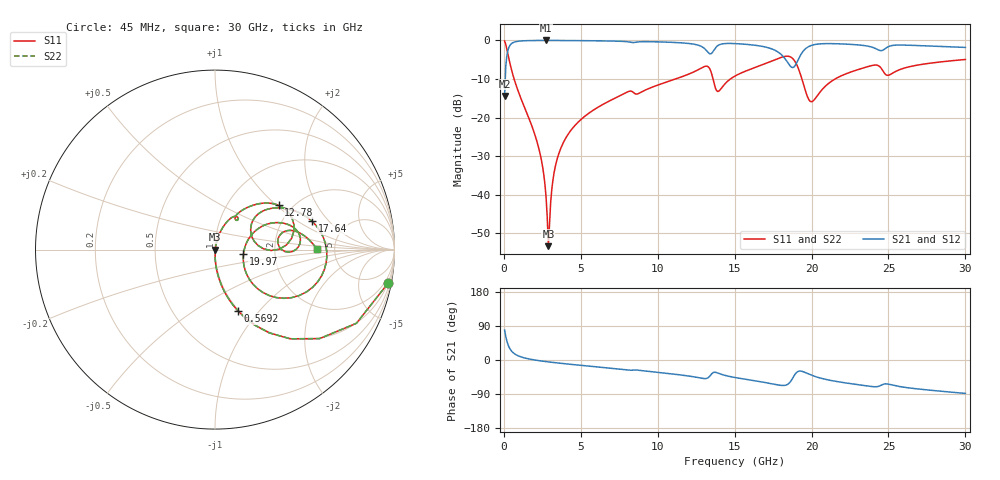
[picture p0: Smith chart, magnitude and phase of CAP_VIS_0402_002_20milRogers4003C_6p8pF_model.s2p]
! S-parameter model data by Modelithics Inc.  support@modelithics.com  813-866-6335  Tampa FL USA
! S-Parameter data specifications:
! Substrate: 20-mil Rogers 4003C, substrate thickness, H=0.508mm, Dielectric constant, Er=3.75
! PCB Mounting Pad Footprint: Pad width, PadW=0.50mm , Pad length, PadL=0.50mm , Pad gap, PadG (edge-to-edge)=0.40mm , Reference planes=1.4mm apart
! Created Wed Nov 18 12:49:20 2015
# hz S ma R 50
! 2 Port Network Data from SP1.SP block
! freq  magS11  angS11  magS21  angS21  magS12  angS12  magS22  angS22
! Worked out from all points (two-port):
!   401 points, 45 MHz to 30 GHz, reference 50 ohm
!   highest |S21| = -0.02 dB at 2.741 GHz (marker M1); lowest = -14.4 dB at 45 MHz (marker M2)
!   |S21| within 3 dB of the highest: 236.9 MHz to 13.25 GHz (13.02 GHz wide, 193 % of centre); 19.41 GHz to end of sweep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
!   lowest |S11| = -53.3 dB at 2.891 GHz (marker M3), VSWR 1.00, Z = 50.2 - j0.0637 ohm
!   |S11| at or under -10 dB: 661.8 MHz to 11.16 GHz (10.5 GHz wide, 178 % of centre); 13.59 GHz to 14.72 GHz (1.131 GHz wide, 7.99 % of centre); 19.37 GHz to 21.53 GHz (2.158 GHz wide, 10.6 % of centre)
!   |S22| runs from -53.3 to -0.2 dB; largest |S21 - S12| = 0
!   S11 on the Smith chart (normalised r, x): 45 MHz: 1, -10; 569.2 MHz: 0.99, -0.78; 12.78 GHz: 1.71, +1.03; 17.64 GHz: 2.90, +1.34; 19.97 GHz: 1.37, -0.07; 30 GHz: 3.60, +0.06
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4.5e7  0.9818 -11.0  0.1899 79.0  0.1899 79.0  0.9818 -11.0
2.696625e8  0.6498 -49.9  0.7596 40.1  0.7596 40.1  0.6498 -49.9
5.692125e8  0.3656 -69.4  0.9299 20.5  0.9299 20.5  0.3656 -69.4
2.216738e9  0.04374 -88.9  0.9971 -1.4  0.9971 -1.4  0.04374 -88.9
2.516288e9  0.02299 -88.2  0.9977 -3.1  0.9977 -3.1  0.02299 -88.2
2.74095e9  0.00928 -81.5  0.9978 -4.3  0.9978 -4.3  0.00928 -81.5
2.890725e9  0.002157 -17.1  0.9978 -5.0  0.9978 -5.0  0.002157 -17.1
3.564712e9  0.0339 77.9  0.997 -8.1  0.997 -8.1  0.0339 77.9
5.062462e9  0.09645 73.9  0.9923 -14.3  0.9923 -14.3  0.09645 73.9
1.007992e10  0.267 55.3  0.9557 -33.0  0.9557 -33.0  0.267 55.3
1.277588e10  0.4319 34.8  0.8458 -47.6  0.8458 -47.6  0.4319 34.8
1.330009e10  0.4516 13.2  0.6901 -46.0  0.6901 -46.0  0.4516 13.2
1.389919e10  0.2177 18.9  0.8535 -34.2  0.8535 -34.2  0.2177 18.9
1.50225e10  0.345 38.8  0.9087 -46.3  0.9087 -46.3  0.345 38.8
1.764356e10  0.563 16.2  0.7408 -64.6  0.7408 -64.6  0.563 16.2
1.846732e10  0.6235 -7.0  0.5103 -63.7  0.5103 -63.7  0.6235 -7.0
1.899154e10  0.5046 -32.0  0.495 -34.4  0.495 -34.4  0.5046 -32.0
1.996508e10  0.1606 -9.2  0.8575 -39.6  0.8575 -39.6  0.1606 -9.2
2.003996e10  0.1614 -2.8  0.8672 -40.8  0.8672 -40.8  0.1614 -2.8
2.273591e10  0.4008 21.8  0.883 -63.5  0.883 -63.5  0.4008 21.8
2.505742e10  0.3566 9.6  0.8398 -64.3  0.8398 -64.3  0.3566 9.6
3e10  0.5657 0.5  0.8107 -88.2  0.8107 -88.2  0.5657 0.5
